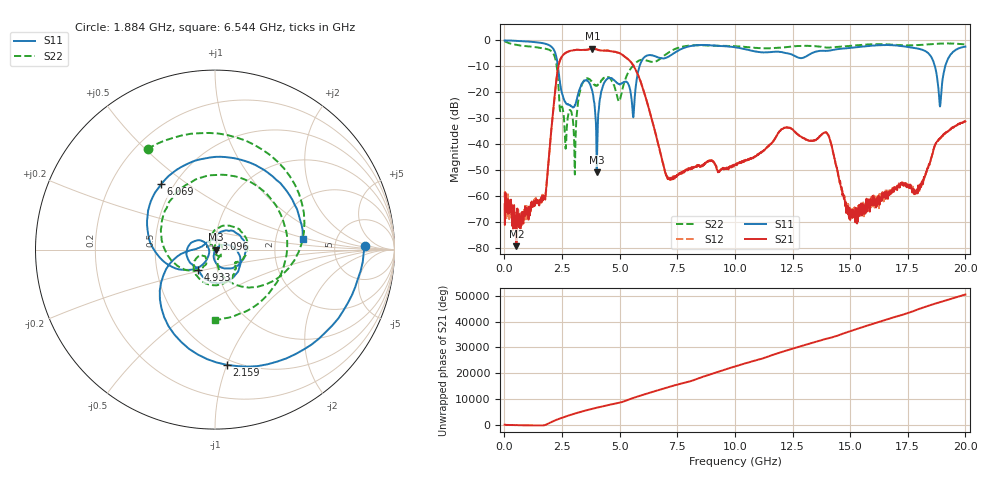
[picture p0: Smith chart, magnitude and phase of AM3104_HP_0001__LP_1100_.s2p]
!Created with skrf (http://scikit-rf.org).
# Hz S RI R 50.0
!freq ReS11 ImS11 ReS21 ImS21 ReS12 ImS12 ReS22 ImS22
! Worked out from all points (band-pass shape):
!   1601 points, 10 MHz to 20 GHz, reference 50 ohm
!   highest |S21| = -3.18 dB at 3.821 GHz (marker M1); lowest = -79.5 dB at 522.2 MHz (marker M2)
!   |S21| within 3 dB of the highest: 2.497 GHz to 5.208 GHz (2.711 GHz wide, 70.4 % of centre)
!   lowest |S11| = -50.9 dB at 4.008 GHz (marker M3), VSWR 1.01, Z = 50.3 - j0.0355 ohm
!   |S11| at or under -10 dB: 2.324 GHz to 5.863 GHz (3.539 GHz wide, 86.5 % of centre); 18.68 GHz to 19.12 GHz (442.9 MHz wide, 2.34 % of centre)
!   |S22| runs from -51.8 to -0.2 dB; largest |S21 - S12| = 0.0063
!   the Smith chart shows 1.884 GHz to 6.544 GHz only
!   S11 on the Smith chart (normalised r, x): 1.884 GHz: 11, +2; 2.159 GHz: 0.45, -1.00; 3.096 GHz: 1.00, +0.12; 4.933 GHz: 0.81, -0.19; 6.069 GHz: 0.43, +0.40; 6.544 GHz: 2.87, +0.43
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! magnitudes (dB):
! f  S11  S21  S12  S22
! 10 MHz  0.0  -63.3  -60.6  -0.2
! 522.2 MHz  -0.1  -79.5  -67.6  -1.7
! 1.884 GHz  -1.6  -49.6  -50.2  -3.4
! 2.159 GHz  -3.8  -23.3  -23.3  -5.7
! 2.621 GHz  -23.6  -5.0  -5.0  -35.5
! 3.096 GHz  -24.2  -3.6  -3.7  -35.6
! 3.346 GHz  -16.9  -3.7  -3.7  -17.4
! 3.821 GHz  -19.7  -3.2  -3.2  -16.1
! 4.008 GHz  -50.9  -3.5  -3.5  -17.5
! 4.933 GHz  -16.7  -4.7  -4.7  -22.8
! 5.582 GHz  -29.4  -9.5  -9.5  -9.8
! 6.069 GHz  -6.5  -20.3  -20.3  -7.5
! 6.544 GHz  -6.1  -35.5  -35.4  -8.2
! 6.682 GHz  -6.6  -40.3  -40.2  -7.6
! 7.181 GHz  -5.9  -53.8  -53.2  -4.3
! 10.01 GHz  -2.6  -48.2  -47.7  -2.2
! 13.34 GHz  -4.9  -38.8  -38.8  -2.2
! 14.04 GHz  -4.0  -36.4  -36.3  -2.7
! 15.04 GHz  -2.8  -66.9  -68.9  -2.1
! 16.68 GHz  -1.8  -58.6  -58.7  -1.5
! 18.9 GHz  -25.5  -37.7  -37.8  -1.2
! 20 GHz  -2.4  -31.3  -31.2  -1.5
